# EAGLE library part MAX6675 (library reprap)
Thermocouple amplifier and A to D converter
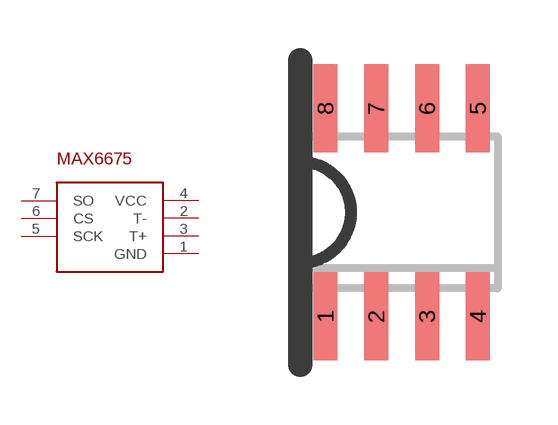
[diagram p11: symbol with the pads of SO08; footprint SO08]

Designator prefix -

## MAX6675  [SO08]
1  GND  pwr
2  T-  in
3  T+  in
4  VCC  pwr
5  SCK  in
6  CS  in
7  SO  out

## Footprint SO08 (pad centres in mm)
SMALL OUTLINE INTEGRATED CIRCUIT body 3.9 mm/JEDEC MS-012AA
smd 0.6 x 2.2: 1 -1.905,-2.6; 2 -0.635,-2.6; 3 0.635,-2.6; 4 1.905,-2.6; 5 1.905,2.6; 6 0.635,2.6; 7 -0.635,2.6; 8 -1.905,2.6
